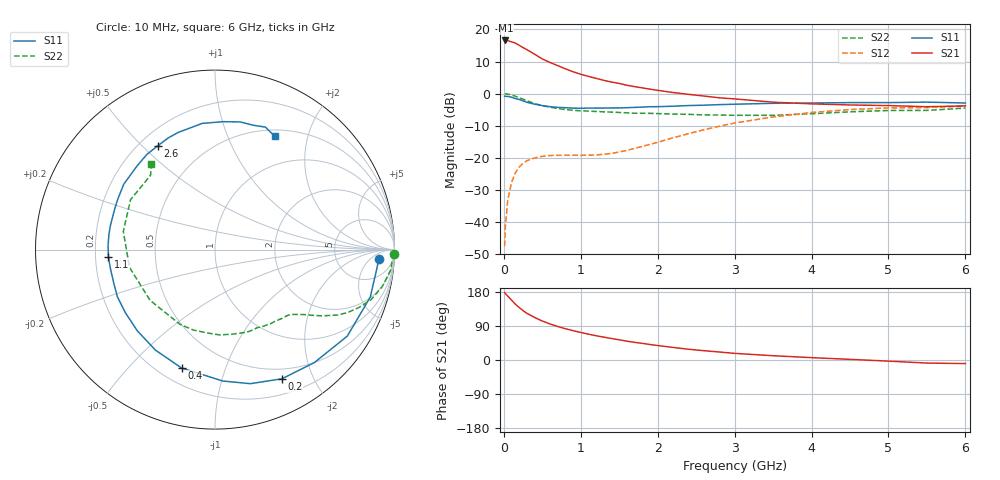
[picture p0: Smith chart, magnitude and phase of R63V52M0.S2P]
! SIEMENS Small Signal Semiconductors
! BFR193
! Si NPN RF Bipolar Junction Transistor in SOT23
! VCE = 3.5 V  IC = 2 mA
! Common Emitter S-Parameters:  May  1996
# GHz  S  MA  R  50
!  f  S11  S21  S12  S22
! GHz  MAG  ANG  MAG  ANG  MAG  ANG  MAG  ANG
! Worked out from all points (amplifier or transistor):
!   36 points, 10 MHz to 6 GHz, reference 50 ohm
!   highest |S21| = 16.6 dB at 20 MHz (marker M1)
!   |S21| within 3 dB of that: start of sweep to 309.7 MHz
!   unconditionally stable (mu >= 1): 1.159 GHz to 2.039 GHz
!   at 250 MHz: K = 0.23, MSG = 18.0 dB, |S12| = -21.7 dB
!   at 1.4 GHz: K = 1.12, MAG = 9.1 dB, |S12| = -18.7 dB
!   at 6 GHz: K = 1.00, MSG = 0.0 dB, |S12| = -3.9 dB
!   S11 on the Smith chart (normalised r, x): 10 MHz: 15, -10; 200 MHz: 0.38, -1.58; 400 MHz: 0.29, -0.72; 1.1 GHz: 0.25, -0.03; 2.6 GHz: 0.27, +0.56; 6 GHz: 0.58, +1.49
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0.01  0.9138 -3.4  6.618 178.1  0.0042 91.9  0.9974 -1.3
0.02  0.9077 -6.8  6.741 175.4  0.0084 85.8  0.9903 -2.6
0.05  0.9046 -17.0  6.701 168.8  0.0216 81.2  0.9862 -6.5
0.1  0.8807 -33.2  6.413 158.1  0.0413 72.3  0.9552 -12.4
0.15  0.8382 -48.7  6.13 147.1  0.0586 63.8  0.9125 -17.9
0.2  0.8107 -62.6  5.666 138.4  0.0718 57.1  0.8644 -21.9
0.25  0.7726 -75.2  5.213 130.3  0.0823 51.9  0.8191 -25.3
0.3  0.7335 -86.6  4.849 123.2  0.0902 47.3  0.7759 -28.0
0.4  0.6854 -105.8  4.115 112.3  0.0996 40.5  0.7006 -31.8
0.5  0.6509 -120.7  3.472 102.9  0.1054 36.2  0.6507 -34.2
0.6  0.626 -133.8  3.064 95.1  0.1087 33.6  0.6159 -36.0
0.7  0.6107 -144.9  2.734 88.4  0.1094 32.6  0.5881 -37.9
0.9  0.5943 -161.6  2.192 77.5  0.1096 33.8  0.549 -41.6
1.1  0.5952 -176.0  1.856 68.2  0.11 37.5  0.5345 -45.9
1.3  0.5971 171.8  1.611 60.3  0.1137 43.7  0.5203 -50.4
1.6  0.6041 156.9  1.351 49.7  0.1309 54.0  0.5027 -58.8
2.2  0.6369 133.1  1.041 33.1  0.2051 63.6  0.4807 -78.7
2.6  0.6604 118.9  0.918 24.6  0.2739 61.7  0.4662 -95.6
3.5  0.7068 95.8  0.736 11.3  0.4335 46.5  0.459 -142.0
4.5  0.7252 78.8  0.666 1.7  0.5654 25.6  0.5207 168.8
5.5  0.7379 67.6  0.625 -8.1  0.6061 6.3  0.5482 130.9
6  0.7143 62.3  0.645 -9.4  0.6396 1.0  0.5955 126.5
